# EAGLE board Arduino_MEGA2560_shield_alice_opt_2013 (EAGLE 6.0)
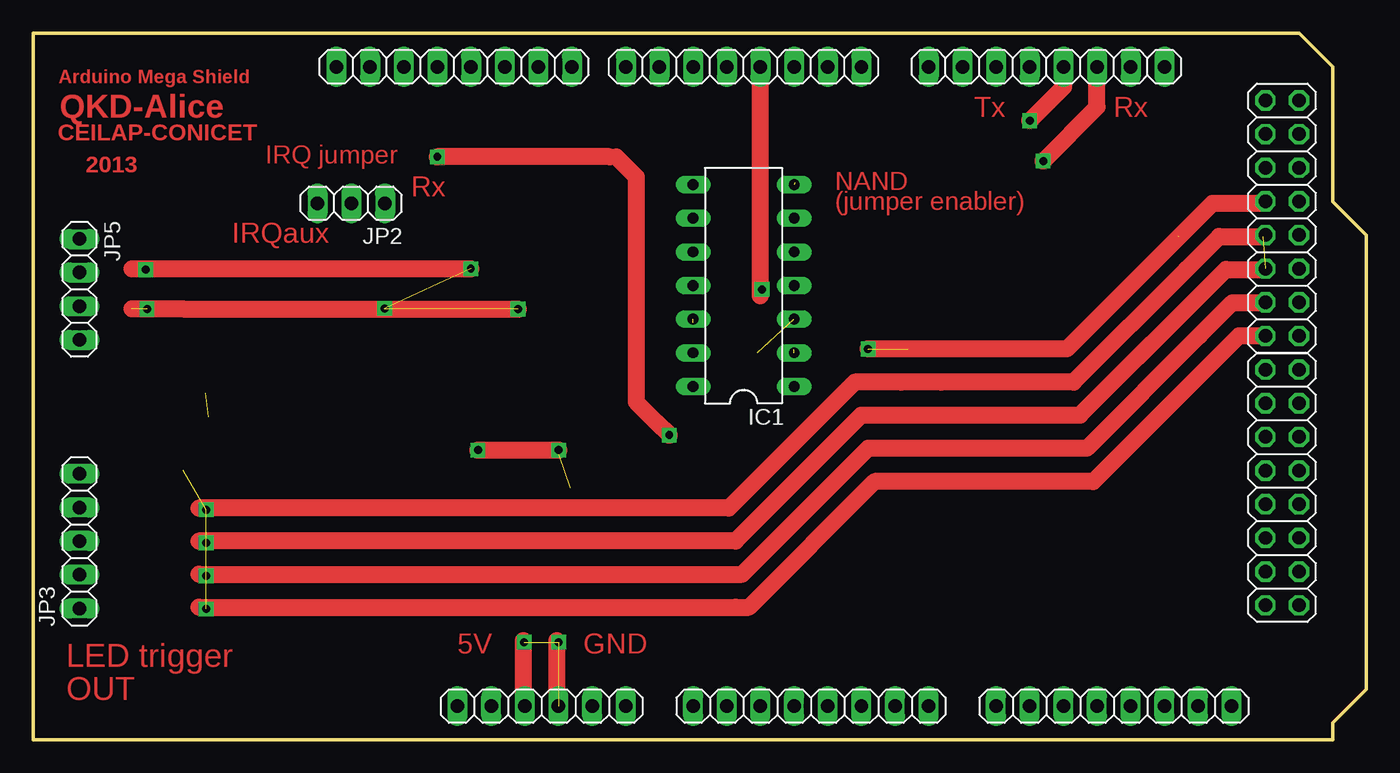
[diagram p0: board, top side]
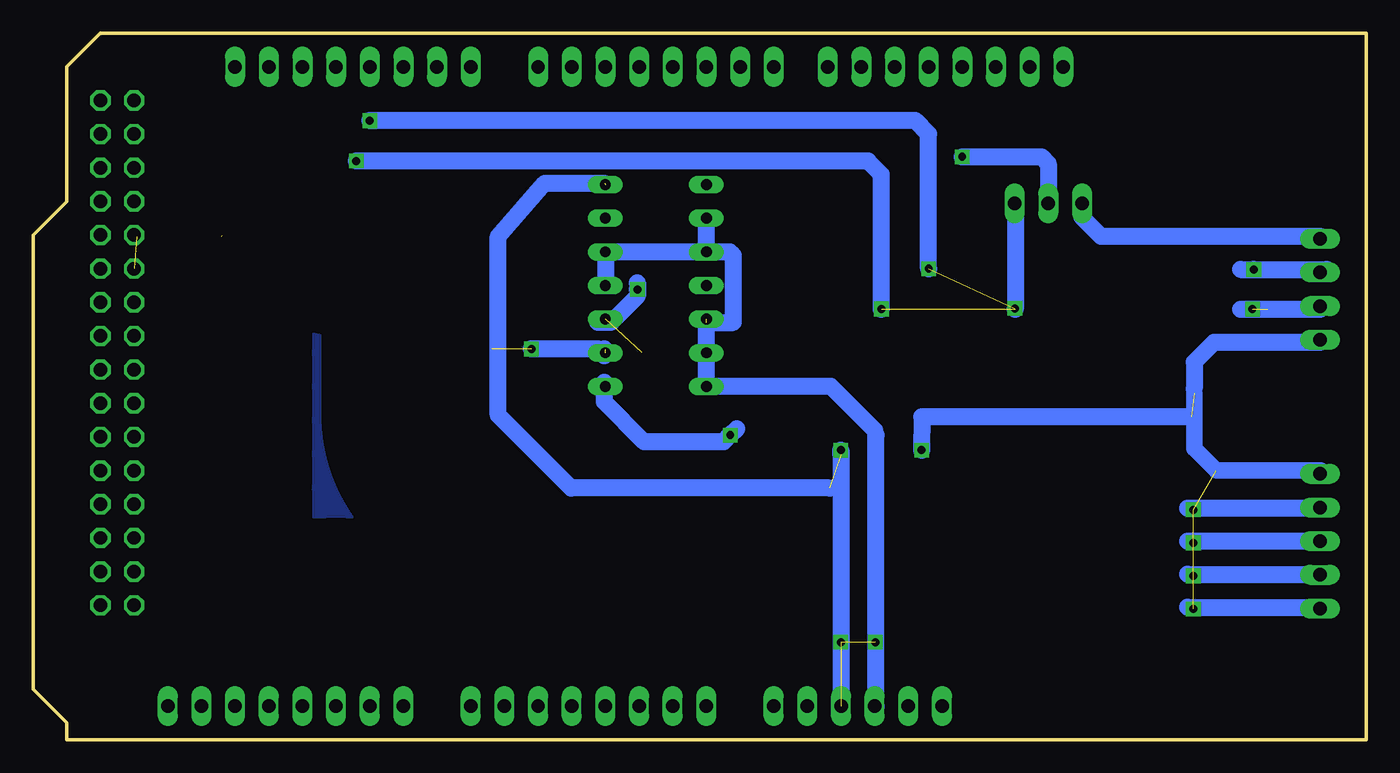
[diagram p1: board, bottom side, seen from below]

Size 100.6 x 53.34 mm. Coordinates in mm from the lower left corner, seen from the top.
Outline: 0,53.34 95.52,53.34 98.06,50.8 98.06,40.64 100.6,38.1 100.6,3.81 98.06,1.27 98.06,0 0,0 0,53.34
Copper layers (1*16): Top 0.035mm / dielectric 1.5mm / Bottom 0.035mm
Design rules: minimum track width 6mil, minimum drill 12mil, track to track 40mil, track to pad 20mil, pad to pad 10mil, via to via 6mil, smd to smd 6mil, copper to edge 50mil, drill to drill 12mil, minimum pad ring 10mil, minimum via ring 10mil, stop-mask expansion 5mil, vias tented up to drill 1mil, thermal gap 10mil
Net classes: 0 default: width 0.152 mm, drill 0.305 mm, clearance 0.152 mm

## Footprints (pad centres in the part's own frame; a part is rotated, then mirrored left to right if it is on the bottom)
1X08 = drill 1.016 long: 1 -8.89,0; 2 -6.35,0; 3 -3.81,0; 4 -1.27,0; 5 1.27,0; 6 3.81,0; 7 6.35,0; 8 8.89,0
DIL14 = drill 0.813 long: 1 -7.62,-3.81; 2 -5.08,-3.81; 3 -2.54,-3.81; 4 0,-3.81; 5 2.54,-3.81; 6 5.08,-3.81; 7 7.62,-3.81; 8 7.62,3.81; 9 5.08,3.81; 10 2.54,3.81; 11 0,3.81; 12 -2.54,3.81; 13 -5.08,3.81; 14 -7.62,3.81
1X03 = drill 1.016 long: 1 -2.54,0; 2 0,0; 3 2.54,0
1X05 = drill 1.016 long: 1 -5.08,0; 2 -2.54,0; 3 0,0; 4 2.54,0; 5 5.08,0
1X04 = drill 1.016 long: 1 -3.81,0; 2 -1.27,0; 3 1.27,0; 4 3.81,0
1X06 = drill 1.016 long: 1 -6.35,0; 2 -3.81,0; 3 -1.27,0; 4 1.27,0; 5 3.81,0; 6 6.35,0
2X08 = drill 1.016 octagon: 1 -8.89,-1.27; 2 -8.89,1.27; 3 -6.35,-1.27; 4 -6.35,1.27; 5 -3.81,-1.27; 6 -3.81,1.27; 7 -1.27,-1.27; 8 -1.27,1.27; 9 1.27,-1.27; 10 1.27,1.27; 11 3.81,-1.27; 12 3.81,1.27; 13 6.35,-1.27; 14 6.35,1.27; 15 8.89,-1.27; 16 8.89,1.27

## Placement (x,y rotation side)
ADCH  [1X08]  81.55,2.54 0 top
ADCL  [1X08]  58.69,2.54 0 top
COMMUNICATION  [1X08]  76.47,50.8 180 top
IC1  74ACT00N  [DIL14]  53.61,34.29 90 top
JP2  [1X03]  24,40.5 180 top
JP3  [1X05]  3.5,15 90 top
JP5  [1X04]  3.5,34 270 top
POWER  [1X06]  38.37,2.54 0 top
PWMH  [1X08]  31.77,50.8 180 top
PWML  [1X08]  53.61,50.8 180 top
XIOH  [2X08]  94.25,39.37 90 top
XIOL  [2X08]  94.25,19.05 90 top

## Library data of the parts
ADCH ADCL COMMUNICATION JP2 JP3 JP5 POWER PWMH PWML XIOH XIOL = pinhead
IC1 = 74xx-eu

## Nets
GND: IC1.7 POWER.4
N$3: XIOL.3
N$7: JP2.3
N$8: IC1.2
N$9: COMMUNICATION.4
N$10: COMMUNICATION.3 JP2.1
N$11: PWML.4
N$14: IC1.4 IC1.5 IC1.9 IC1.10 IC1.12 IC1.13 IC1.14
S$5: XIOL.10
S$8: JP3.3
S$23: XIOH.6
S$27: IC1.3

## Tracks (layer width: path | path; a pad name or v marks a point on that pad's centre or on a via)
GND  (via drill 0.6)  (9 unrouted)
  Top 1.27: v33.56,21.87 v39.66,21.87
  Bottom 1.24: 3.45,20.32 11.32,20.32 13,22 13,26.19
  Bottom 1.27: POWER.4 39.66,21.56 v39.66,21.87 | v33.56,21.87 33.54,24.38 13.22,24.38 | 57.5,42 62,42 65.5,38 65.5,24.5 60,19 40.5,19
  other vias: 13.06,17.37 13.06,14.87 13.06,12.37 13.06,9.87 37.06,7.37 39.66,7.37
N$1
  Top 1.27: 44,44 45.5,42.5 45.5,25.5 47,24 48,23
N$7
  Top 1.27: 21.46,39.96 JP2.3
N$8  (1 unrouted)
N$9  (via drill 0.6)  (1 unrouted)
  Top 1.27: 7.45,35.56 v33.03,35.56 | v75.2,46.74 77.74,49.28 COMMUNICATION.4
  Bottom 1.27: v33.03,35.56 33.03,45.72 34.04,46.74 v75.2,46.74
  other vias: 26.53,32.56
N$10  (via drill 0.6)  (2 unrouted)
  Top 1.27: 7.45,32.52 11.45,32.51 v36.59,32.51 | v76.22,43.69 80.28,47.75 COMMUNICATION.3
  Bottom 1.27: v36.59,32.51 36.59,42.67 37.61,43.69 v76.22,43.69 | JP2.1 26.5,40.46 26.5,32.51
  other vias: 8.59,32.51
N$11
  Top 1.27: 54.88,33.51 PWML.4
N$14  (1 unrouted)
  Bottom 1.27: 37.11,23.37 40.41,26.67 IC1.14 IC1.13 49.8,31.5 47.77,31.5 47.77,36.58 48.02,36.83 IC1.10 | IC1.10 IC1.5 IC1.4 | IC1.10 IC1.9
S$1
  Top 1.27: 65.5,27 78.5,27 87,35.5 89.5,38 93,38
S$2
  Top 1.27: 87.5,33 79,24.5 62.5,24.5 53,15 12.5,15
S$3
  Top 1.27: 12.5,12.5 53.5,12.5 63,22 79.5,22 88,30.5 90.5,33 93,33
S$4
  Bottom 1.27: 13.5,17.5 3,17.5
S$6
  Top 1.27: 68.5,27 62,27 52.5,17.5 12.5,17.5
S$7
  Top 1.27: 12.5,10 53,10 | 53,10 | 53,10 54,10 63.5,19.5 80,19.5 80.5,20 | 88.5,28 80.5,20 | 80.5,20 | 80.5,20 91,30.5 93,30.5
S$8
  Bottom 1.27: 13.5,15 JP3.3
S$9
  Bottom 1.27: 13.5,12.5 3.5,12.5
S$10
  Bottom 1.27: 13.5,10 3,10
S$11
  Bottom 1.27: 37,2.5 37,23
S$12
  Top 1.27: 37,2.5 37,7.5
S$13
  Top 1.27: 39.5,7.5 39.5,2.5
S$14
  Bottom 1.27: 3.5,30 11.5,30 13,28.5 13,26.5
S$15
  Bottom 1.27: 3.5,38 20,38 21.5,39.5 21.5,40.5
S$16
  Bottom 1.27: 9.5,32.5 3.5,32.5
S$17  (via drill 0.6)
  Bottom 1.27: 9.5,35.5 v8.5,35.5 3,35.5
S$18  (via drill 0.6)
  Bottom 1.27: 47.5,23.5 v48,23 48.5,22.5 54.5,22.5 57.5,25.5 57.5,27
S$19  (via drill 0.6)
  Top 1.27: 43.5,44 v30.5,44
  Bottom 1.27: v30.5,44 24.5,44 24,43.5 24,40
S$20  (via drill 0.6)
  Bottom 1.27: 55,34.5 v55,34 55,33.5 57,31.5 58,31.5
S$21
  pour Bottom (isolate 12.7): 0,53 95.5,53 98,50.5 98,40.5 100.5,38 100.5,4 98,1.5 98,0 0,0
S$22
  pour Top (isolate 12.7): 0,53 95.5,53 95.5,53 98,50.5 98,40.5 100.5,38 100.5,4 98,1.5 98,0 0,0
S$23  (1 unrouted)
S$24  (1 unrouted)
S$25  (via drill 0.6)  (1 unrouted)
  Top 1.27: 93,40.5 89,40.5 78,29.5 v63,29.5
  Bottom 1.27: 57.5,29.5 57.5,29 58,29.5 v63,29.5
S$26
  Top 1.27: 79,24.5 90,35.5 93,35.5
S$27  (1 unrouted)

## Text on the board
Top: Arduino Mega Shield | QKD-Alice | Tx | Rx | CEILAP-CONICET | 2013 | IRQ jumper | Rx | NAND | (jumper enabler) | IRQaux | 5V | GND | LED trigger | OUT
